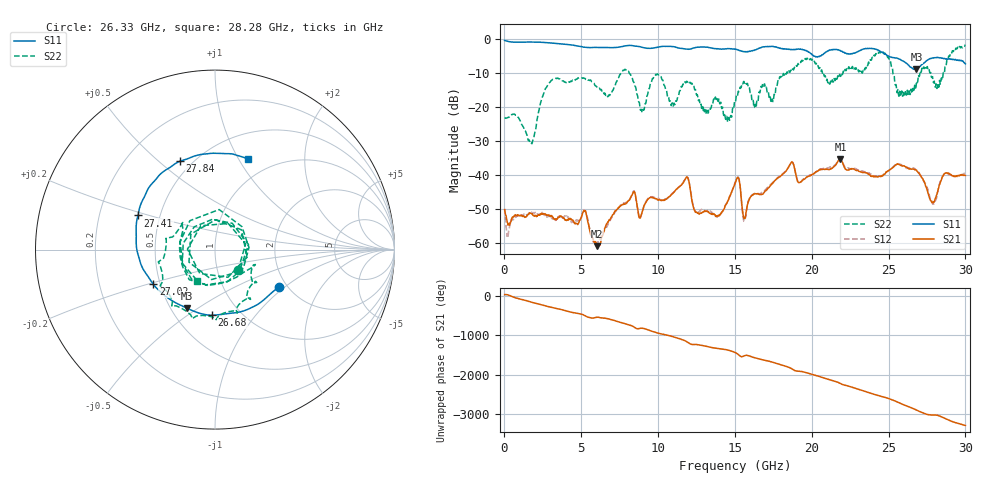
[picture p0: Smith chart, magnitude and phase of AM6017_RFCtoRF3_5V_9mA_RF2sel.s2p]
!Agilent Technologies,E8364B,MY43040894,A.07.50.67
!Agilent E8364B: A.07.50.67
!Date: Tuesday, August 21, 2018 13:42:00
!Correction: S11(Full 2 Port(1,2))
!S21(Full 2 Port(1,2))
!S12(Full 2 Port(1,2))
!S22(Full 2 Port(1,2))
!S2P File: Measurements: S11, S21, S12, S22:
# Hz S  dB  R 50
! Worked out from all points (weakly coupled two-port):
!   1601 points, 10 MHz to 30 GHz, reference 50 ohm
!   highest |S21| = -35.32 dB at 21.87 GHz (marker M1); lowest = -61.0 dB at 6.027 GHz (marker M2)
!   lowest |S11| = -8.8 dB at 26.81 GHz (marker M3), VSWR 2.14, Z = 30.2 - j22.7 ohm
!   |S11| at or under -10 dB: nowhere
!   |S22| runs from -30.8 to -1.6 dB; largest |S21 - S12| = 0.0063
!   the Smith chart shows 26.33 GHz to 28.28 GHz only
!   S11 on the Smith chart (normalised r, x): 26.33 GHz: 1.81, -0.91; 26.68 GHz: 0.74, -0.63; 27.02 GHz: 0.46, -0.21; 27.41 GHz: 0.38, +0.18; 27.84 GHz: 0.43, +0.59; 28.28 GHz: 0.77, +1.10
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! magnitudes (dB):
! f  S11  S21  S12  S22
! 10 MHz  -0.3  -50.2  -49.9  -23.1
! 1.753 GHz  -0.8  -51.3  -51.1  -30.6
! 2.934 GHz  -1.1  -52.0  -52.1  -12.8
! 5.015 GHz  -2.2  -52.3  -52.3  -11.3
! 6.027 GHz  -2.4  -61.0  -60.1  -14.1
! 7.957 GHz  -1.9  -48.2  -48.0  -9.0
! 8.97 GHz  -2.4  -50.8  -50.9  -21.6
! 10.02 GHz  -2.3  -47.3  -46.9  -10.5
! 13.88 GHz  -2.8  -52.0  -52.2  -18.1
! 15.01 GHz  -2.9  -42.6  -42.3  -18.4
! 15.62 GHz  -3.7  -52.8  -53.5  -12.9
! 20.01 GHz  -4.5  -39.9  -39.9  -6.1
! 21.87 GHz  -3.3  -35.3  -35.0  -10.9
! 25.01 GHz  -5.0  -38.7  -38.7  -5.5
! 26.33 GHz  -7.7  -38.2  -38.0  -15.4
! 26.68 GHz  -8.7  -38.4  -38.1  -14.0
! 26.81 GHz  -8.8  -38.7  -38.5  -12.7
! 27.02 GHz  -8.1  -39.7  -39.6  -10.6
! 27.41 GHz  -6.6  -43.3  -42.6  -7.9
! 27.84 GHz  -5.5  -48.2  -48.1  -11.1
! 28.28 GHz  -5.4  -43.4  -43.4  -14.0
! 30 GHz  -7.2  -40.1  -39.3  -1.6
